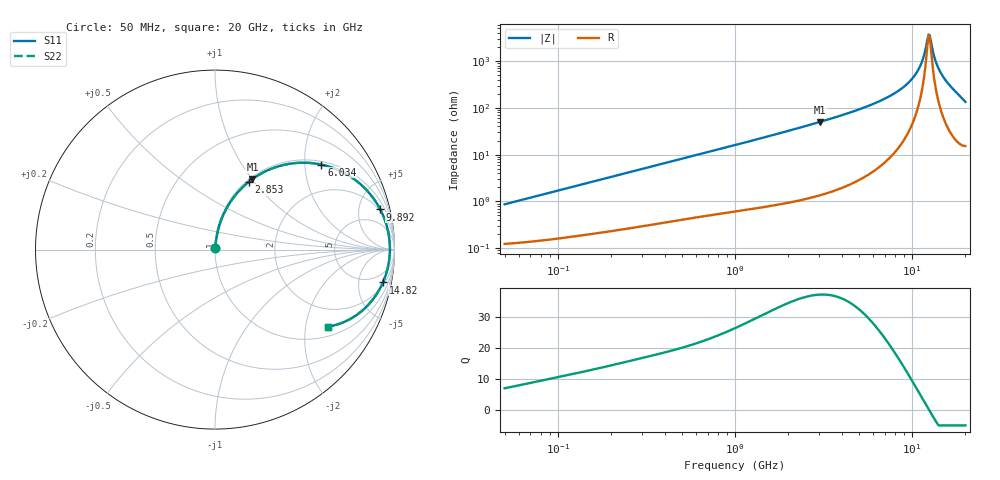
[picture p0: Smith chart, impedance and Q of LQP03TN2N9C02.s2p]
!Murata Part Number: LQP03TN2N9C02
!These Parameters are Measured in Series Mode Connection
!  o--[Z]--o
!Port1  Port2
!  o-------o
!Freq. Start=50[MHz] Stop=20[GHz], 401[Steps]
# Hz S RI R 50
!Freq.(Hz) S11(Real) S11(Imag) S21(Real) S21(Imag) S12(Real) S12(Imag) S22(Real) S22(Imag)
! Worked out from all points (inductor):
!   401 points, 50 MHz to 20 GHz, reference 50 ohm
!   read as one part in series: L = 2.72 nH near 51.52 MHz
!   highest Q = 37.1 at 3.03 GHz (marker M1), where L = 2.64 nH
!   self-resonance near 12.38 GHz
!   S11 on the Smith chart (normalised r, x): 50 MHz: 1.00, +0.02; 2.853 GHz: 1.03, +0.94; 6.034 GHz: 1.09, +2.43; 9.892 GHz: 1.81, +7.94; 14.82 GHz: 2, -10; 20 GHz: 1.31, -2.66
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5e7  0.0013 0.00856  0.9987 -0.00856  0.9987 -0.00856  0.0013 0.00856
1.364002e8  0.00239 0.0228  0.9976 -0.0228  0.9976 -0.0228  0.00239 0.0228
3.721004e8  0.00698 0.06  0.993 -0.06  0.993 -0.06  0.00698 0.06
1e9  0.0305 0.154  0.9695 -0.154  0.9695 -0.154  0.0305 0.154
1.766834e9  0.0812 0.2584  0.9188 -0.2584  0.9188 -0.2584  0.0812 0.2584
2.728004e9  0.1739 0.3657  0.8261 -0.3657  0.8261 -0.3657  0.1739 0.3657
2.853386e9  0.188 0.3774  0.812 -0.3774  0.812 -0.3774  0.188 0.3774
3.029571e9  0.2083 0.3928  0.7917 -0.3928  0.7917 -0.3928  0.2083 0.3928
4.539627e9  0.4006 0.4756  0.5994 -0.4756  0.5994 -0.4756  0.4006 0.4756
6.034176e9  0.593 0.4736  0.407 -0.4736  0.407 -0.4736  0.593 0.4736
7.442007e9  0.7476 0.4112  0.2524 -0.4112  0.2524 -0.4112  0.7476 0.4112
8.774992e9  0.8578 0.317  0.1422 -0.317  0.1422 -0.317  0.8578 0.317
9.892087e9  0.9209 0.2238  0.0791 -0.2238  0.0791 -0.2238  0.9209 0.2238
1.115139e10  0.9619 0.1133  0.0381 -0.1133  0.0381 -0.1133  0.9619 0.1133
1.166392e10  0.9702 0.0684  0.0298 -0.0684  0.0298 -0.0684  0.9702 0.0684
1.220001e10  0.9743 0.0223  0.0257 -0.0223  0.0257 -0.0223  0.9743 0.0223
1.238412e10  0.9746 0.00667  0.0254 -0.00667  0.0254 -0.00667  0.9746 0.00667
1.276073e10  0.9737 -0.0248  0.0263 0.0248  0.0263 0.0248  0.9737 -0.0248
1.375312e10  0.962 -0.1042  0.038 0.1042  0.038 0.1042  0.962 -0.1042
1.482269e10  0.9357 -0.1829  0.0643 0.1829  0.0643 0.1829  0.9357 -0.1829
1.696185e10  0.8465 -0.3156  0.1535 0.3156  0.1535 0.3156  0.8465 -0.3156
2e10  0.6281 -0.4293  0.3719 0.4293  0.3719 0.4293  0.6281 -0.4293
